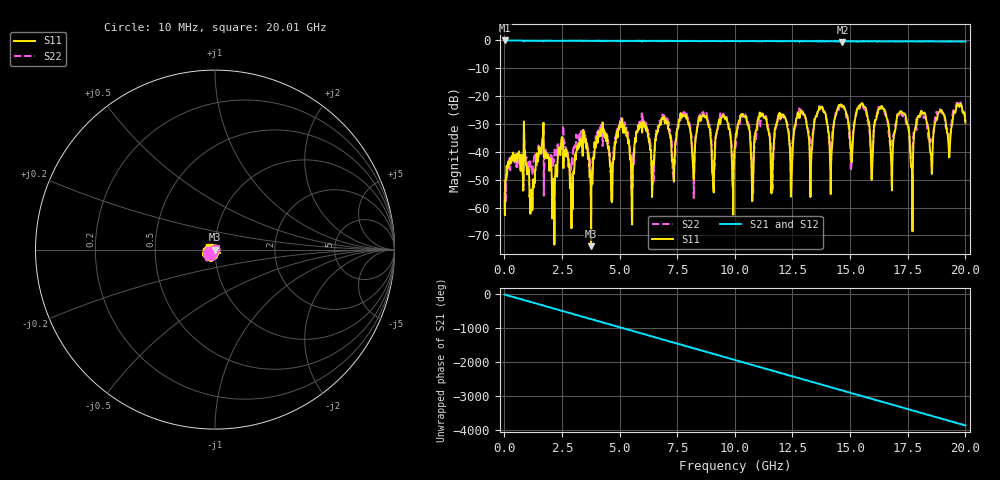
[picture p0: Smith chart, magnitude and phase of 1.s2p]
! 1/20/2025 12:56:29 PM
! D:\YHJ\ZDC25-30C0.5-18G-656\1.S2P
! CHANNEL.1
! TR.MEASUREMENT
! CORRECTED.DATA
! RF.CORRECTION: FULL.TWO.PORT.CAL.PORT.1.2
! AVERAGING.OFF
! IF.BANDWIDTH: NO.IFBW
! SWEEPTYPE:  FREQ.SWEEP(Linear)
! Reference Plane Port Info
! PORT:  PORT1  PORT2
! DISTANCE:  0  m  0  m
! TIME:  0  s  0  s
! PHASE.OFFSET:  0 °  0 °
! LOSS:  0  dB  0  dB
! REF.LOSS:  0  dB  0  dB
! REF.FREQ:  0  Hz  0  Hz
! Power Info
! POWER:  -10  dBm  -10  dBm
! EFF.POWER:  -10  dBm  -10  dBm
! SOURCE.ATTEN:  0  dB  0  dB
! TEST.ATTEN:  0  dB  0  dB
# GHZ S RI R 50.0
! FREQ.GHZ  S11RE  S11IM  S21RE  S21IM  S12RE  S12IM  S22RE  S22IM
!; PortSelection: Port_12
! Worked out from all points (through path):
!   1482 points, 10 MHz to 20.01 GHz, reference 50 ohm
!   highest |S21| = -0.01 dB at 23.5 MHz (marker M1); lowest = -0.5 dB at 14.67 GHz (marker M2)
!   group delay of S21, straight-line fit = 537 ps
!   lowest |S11| = -73.9 dB at 3.763 GHz (marker M3), VSWR 1.00, Z = 50 + j0.0145 ohm
!   |S11| at or under -10 dB: start of sweep to end of sweep
!   |S22| runs from -58.3 to -22.3 dB; largest |S21 - S12| = 0.035
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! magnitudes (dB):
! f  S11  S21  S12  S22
! 10 MHz  -57.5  0.0  0.0  -57.0
! 23.5 MHz  -62.8  0.0  0.0  -52.8
! 1.185 GHz  -53.5  -0.1  -0.1  -46.5
! 1.603 GHz  -40.1  -0.1  -0.1  -37.5
! 2.926 GHz  -53.8  -0.1  -0.1  -42.6
! 3.345 GHz  -37.9  -0.1  -0.1  -35.0
! 3.763 GHz  -73.9  -0.1  -0.1  -47.4
! 4.223 GHz  -32.9  -0.2  -0.1  -31.8
! 4.668 GHz  -58.1  -0.2  -0.2  -48.0
! 5.033 GHz  -29.2  -0.3  -0.3  -28.8
! 5.532 GHz  -65.2  -0.2  -0.2  -48.2
! 6.68 GHz  -31.2  -0.2  -0.2  -31.3
! 10.01 GHz  -36.9  -0.2  -0.2  -39.1
! 11.16 GHz  -26.4  -0.3  -0.3  -26.8
! 11.62 GHz  -48.1  -0.2  -0.3  -45.1
! 12.01 GHz  -26.6  -0.3  -0.2  -27.2
! 12.46 GHz  -50.4  -0.3  -0.2  -38.0
! 12.93 GHz  -25.7  -0.4  -0.2  -26.4
! 13.35 GHz  -39.1  -0.3  -0.3  -36.7
! 14.67 GHz  -23.3  -0.5  -0.3  -23.7
! 16.68 GHz  -31.3  -0.3  -0.3  -33.7
! 20.01 GHz  -29.6  -0.4  -0.4  -29.0
